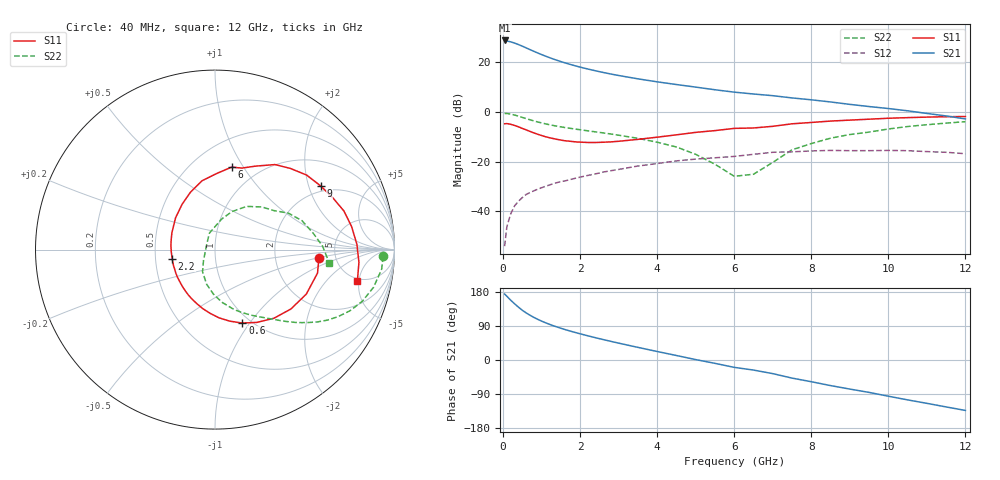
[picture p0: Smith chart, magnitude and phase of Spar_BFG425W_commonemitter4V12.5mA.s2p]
! Filename: 412bfg425.001
! BFG425W Field C1
! V1=8.355E-001V,V2=4.000E+000V, I1=1.439E-004A, I2=1.249E-002A
# GHz  S  MA  R 50
!  S11  S21  S12  S22
!Freq(GHz)  Mag  Ang  Mag  Ang  Mag  Ang  Mag  Ang
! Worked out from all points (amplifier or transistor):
!   44 points, 40 MHz to 12 GHz, reference 50 ohm
!   highest |S21| = 28.8 dB at 40 MHz (marker M1)
!   |S21| within 3 dB of that: start of sweep to 600.2 MHz
!   unconditionally stable (mu >= 1): start of sweep to 46.57 MHz; 1.688 GHz to end of sweep
!   at 700 MHz: K = 0.62, MSG = 28.8 dB, |S12| = -32.4 dB
!   at 2.4 GHz: K = 1.13, MAG = 18.6 dB, |S12| = -24.9 dB
!   at 12 GHz: K = 1.37, MAG = 3.3 dB, |S12| = -16.8 dB
!   S11 on the Smith chart (normalised r, x): 40 MHz: 3.70, -0.52; 600 MHz: 0.91, -0.92; 2.2 GHz: 0.61, -0.07; 6 GHz: 0.75, +0.89; 9 GHz: 1.80, +2.41; 12 GHz: 4.70, -4.76
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0.04  0.581 -4.6  27.57 174.1  0.002 44.3  0.937 -2.3
0.2  0.566 -26.0  25.85 157.6  0.009 70.7  0.908 -13.4
0.3  0.537 -38.0  24.39 148.2  0.013 68.1  0.87 -19.3
0.4  0.504 -49.4  22.8 139.4  0.016 65.1  0.826 -24.4
0.5  0.468 -60.1  21.17 131.1  0.019 61.8  0.78 -28.7
0.6  0.437 -69.6  19.52 124.2  0.022 59.7  0.737 -32.3
0.8  0.381 -86.6  16.66 112.4  0.026 56.2  0.662 -37.8
0.9  0.357 -94.1  15.43 107.3  0.028 54.9  0.631 -40.1
1  0.337 -101.3  14.33 102.6  0.03 53.9  0.604 -42.2
1.2  0.305 -114.4  12.48 94.4  0.034 52.2  0.557 -45.8
1.4  0.282 -126.4  11 87.2  0.038 50.9  0.519 -48.9
1.6  0.265 -138.0  9.808 80.7  0.041 49.7  0.489 -51.8
2.2  0.244 -168.1  7.341 63.9  0.053 45.4  0.419 -60.8
3  0.258 158.5  5.438 44.5  0.07 37.7  0.342 -73.6
3.5  0.282 141.2  4.658 33.3  0.082 31.9  0.296 -82.5
4.5  0.348 113.1  3.577 11.9  0.104 18.5  0.198 -103.7
6  0.469 78.6  2.514 -19.4  0.128 -5.2  0.051 167.6
6.5  0.478 71.8  2.308 -26.6  0.141 -7.9  0.056 143.9
8.5  0.658 39.1  1.596 -67.5  0.169 -44.7  0.298 53.9
9  0.688 30.9  1.427 -76.7  0.167 -53.1  0.353 42.3
10.5  0.772 9.5  1.059 -105.2  0.167 -80.4  0.511 18.4
12  0.812 -12.3  0.726 -133.1  0.145 -110.9  0.64 -6.5
